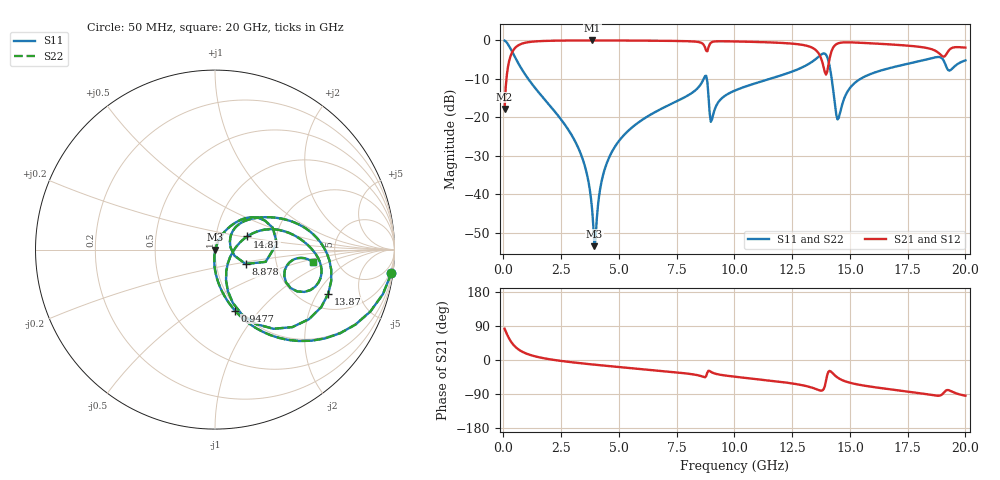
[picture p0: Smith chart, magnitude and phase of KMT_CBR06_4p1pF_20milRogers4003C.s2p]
! Data measured by Modelithics Inc. support@modelithics.com 813-866-6335
! KEMET CBR0603 4.1pF, Pad Width= 0.851mm, Pad Length= 0.64mm, Pad Gap= 0.62mm, 20mil Rogers 4003C substrate Data, January 2022
# hz S ma R 50
! 2 Port Network Data from SP1.SP block
! freq  magS11  angS11  magS21  angS21  magS12  angS12  magS22  angS22
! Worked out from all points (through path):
!   401 points, 50 MHz to 20 GHz, reference 50 ohm
!   highest |S21| = -0.02 dB at 3.841 GHz (marker M1); lowest = -17.8 dB at 50 MHz (marker M2)
!   group delay of S21, straight-line fit = 15.6 ps
!   lowest |S11| = -53.4 dB at 3.94 GHz (marker M3), VSWR 1.00, Z = 50.2 - j0.119 ohm
!   |S11| at or under -10 dB: 1.073 GHz to 8.666 GHz (7.594 GHz wide, 156 % of centre); 8.804 GHz to 11.53 GHz (2.724 GHz wide, 26.8 % of centre); 14.21 GHz to 15.45 GHz (1.243 GHz wide, 8.38 % of centre)
!   |S22| runs from -53.4 to -0.1 dB; largest |S21 - S12| = 0
!   S11 on the Smith chart (normalised r, x): 50 MHz: 1, -15; 947.8 MHz: 0.96, -0.75; 8.878 GHz: 1.39, -0.23; 13.87 GHz: 2.76, -2.50; 14.81 GHz: 1.42, +0.22; 20 GHz: 3.30, -0.66
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5e7  0.9916 -7.6  0.1288 82.4  0.1288 82.4  0.9916 -7.6
3.4925e8  0.7379 -43.5  0.6742 46.4  0.6742 46.4  0.7379 -43.5
9.4775e8  0.3581 -71.8  0.9326 18.0  0.9326 18.0  0.3581 -71.8
3.391625e9  0.03103 -95.5  0.9976 -8.9  0.9976 -8.9  0.03103 -95.5
3.690875e9  0.01412 -93.0  0.9979 -10.8  0.9979 -10.8  0.01412 -93.0
3.8405e9  0.006284 -83.6  0.9979 -11.7  0.9979 -11.7  0.006284 -83.6
3.94025e9  0.002131 -33.7  0.9979 -12.3  0.9979 -12.3  0.002131 -33.7
4.289375e9  0.01675 68.5  0.9976 -14.4  0.9976 -14.4  0.01675 68.5
4.688375e9  0.03542 69.7  0.997 -16.7  0.997 -16.7  0.03542 69.7
6.73325e9  0.1247 60.4  0.989 -28.2  0.989 -28.2  0.1247 60.4
8.678375e9  0.3217 30.2  0.8691 -45.2  0.8691 -45.2  0.3217 30.2
8.877875e9  0.1887 -25.1  0.8112 -28.3  0.8112 -28.3  0.1887 -25.1
9.0275e9  0.09372 27.6  0.9501 -32.8  0.9501 -32.8  0.09372 27.6
1.0025e10  0.2236 44.4  0.9686 -44.1  0.9686 -44.1  0.2236 44.4
1.336662e10  0.5288 12.0  0.8043 -73.1  0.8043 -73.1  0.5288 12.0
1.386538e10  0.6774 -21.2  0.4453 -76.7  0.4453 -76.7  0.6774 -21.2
1.406488e10  0.5487 -53.5  0.4695 -31.5  0.4695 -31.5  0.5487 -53.5
1.446388e10  0.09416 -28.2  0.9096 -46.2  0.9096 -46.2  0.09416 -28.2
1.4813e10  0.1941 22.2  0.9434 -56.6  0.9434 -56.6  0.1941 22.2
1.670825e10  0.436 11.4  0.8881 -77.1  0.8881 -77.1  0.436 11.4
1.905238e10  0.551 -25.3  0.6134 -87.2  0.6134 -87.2  0.551 -25.3
2e10  0.5504 -7.3  0.8057 -94.3  0.8057 -94.3  0.5504 -7.3
